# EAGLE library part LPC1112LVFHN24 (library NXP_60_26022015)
32-bit ARM Cortex-M0 microcontroller The LPC111xLV/LPC11xxLVUK is an ARM Cortex-M0-based, low-cost 32-bit MCU family, designed for 8/16-bit microcontroller applications, offering performance, low power, simple instruction set and memory addressing together with reduced code size compared to existing 8/16-bit architectures. The LPC111xLV/LPC11xxLVUK operate at CPU frequencies of up to 50 MHz. The peripherals of the LPC111xLV/LPC11xxLVUK include up to 32 kB of flash memory, up to 8 kB of SRAM data memory, a Fast-mode Plus I 2 C-bus interface, one SSP/SPI interface, one UART, four general-purpose counter/timers, an 8-bit ADC, and up to 27 general-purpose I/O pins. MK - Datasheet available on www.nxp.com
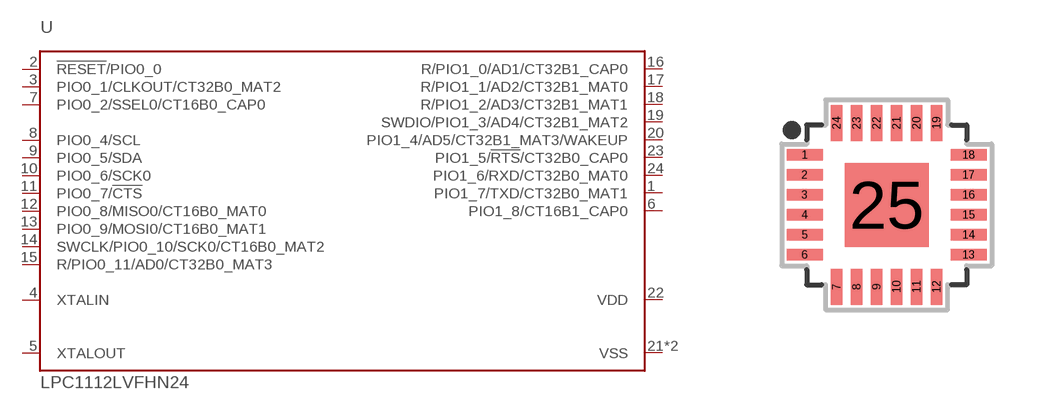
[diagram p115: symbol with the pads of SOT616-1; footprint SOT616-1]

Designator prefix U

## LPC1112LVFHN24  [SOT616-1]
1  PIO1_7/TXD/CT32B0_MAT1
2  !RESET!/PIO0_0
3  PIO0_1/CLKOUT/CT32B0_MAT2
4  XTALIN  in
5  XTALOUT  out
6  PIO1_8/CT16B1_CAP0
7  PIO0_2/SSEL0/CT16B0_CAP0
8  PIO0_4/SCL
9  PIO0_5/SDA
10  PIO0_6/SCK0
11  PIO0_7/!CTS!
12  PIO0_8/MISO0/CT16B0_MAT0
13  PIO0_9/MOSI0/CT16B0_MAT1
14  SWCLK/PIO0_10/SCK0/CT16B0_MAT2
15  R/PIO0_11/AD0/CT32B0_MAT3
16  R/PIO1_0/AD1/CT32B1_CAP0
17  R/PIO1_1/AD2/CT32B1_MAT0
18  R/PIO1_2/AD3/CT32B1_MAT1
19  SWDIO/PIO1_3/AD4/CT32B1_MAT2
20  PIO1_4/AD5/CT32B1_MAT3/WAKEUP
21  VSS  pwr
22  VDD  pwr
23  PIO1_5/!RTS!/CT32B0_CAP0
24  PIO1_6/RXD/CT32B0_MAT0
25  VSS  pwr

## Footprint SOT616-1 (pad centres in mm)
SOT616-1 HVQFN24: plastic thermal enhanced very thin quad flat package; no leads; 24 terminals; body 4 x 4 x 0.85 mm JEDEC: MO-220 IEC: -- JEITA: --
smd 0.9 x 0.29: 1 -2.05,1.25; 2 -2.05,0.75; 3 -2.05,0.25; 4 -2.05,-0.25; 5 -2.05,-0.75; 6 -2.05,-1.25; 13 2.05,-1.25; 14 2.05,-0.75; 15 2.05,-0.25; 16 2.05,0.25; 17 2.05,0.75; 18 2.05,1.25
smd 0.29 x 0.9: 7 -1.25,-2.05; 8 -0.75,-2.05; 9 -0.25,-2.05; 10 0.25,-2.05; 11 0.75,-2.05; 12 1.25,-2.05; 19 1.25,2.05; 20 0.75,2.05; 21 0.25,2.05; 22 -0.25,2.05; 23 -0.75,2.05; 24 -1.25,2.05
smd 2.1 x 2.1: 25 0,0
